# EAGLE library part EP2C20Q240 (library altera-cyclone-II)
EP2C20Q240 Auto generated by make-symbol-device-package-bsdl.ulp Rev. 19 Tip: Use split-device-symbol.ulp to generate a Device with multiple small symbols! Read HELP. Source: EP2C20Q240.BSD
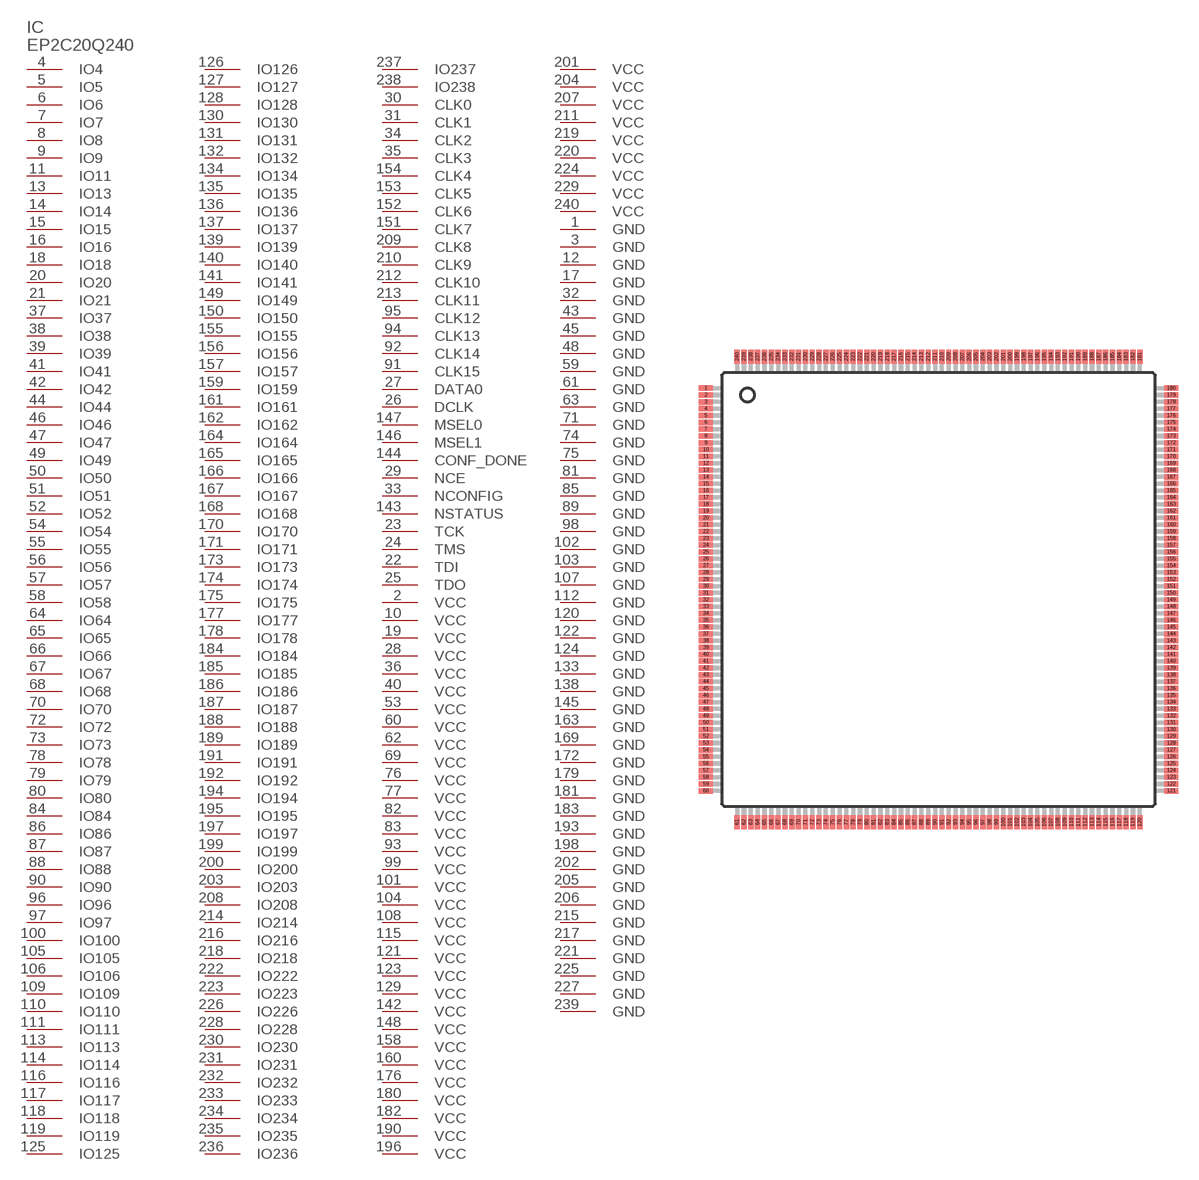
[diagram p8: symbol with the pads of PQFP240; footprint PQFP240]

Designator prefix IC

## EP2C20Q240 (MPN: EP2C20Q240C8N; OC_FARNELL: 1453472; OC_NEWARK: 51R0562)  [PQFP240]
1  GND  pwr
2  VCC  pwr
3  GND  pwr
4  IO4  out
5  IO5  out
6  IO6
7  IO7
8  IO8
9  IO9
10  VCC  pwr
11  IO11
12  GND  pwr
13  IO13
14  IO14
15  IO15
16  IO16
17  GND  pwr
18  IO18
19  VCC  pwr
20  IO20
21  IO21
22  TDI  in
23  TCK  in
24  TMS  in
25  TDO  out
26  DCLK
27  DATA0
28  VCC  pwr
29  NCE  in
30  CLK0
31  CLK1
32  GND  pwr
33  NCONFIG  in
34  CLK2
35  CLK3
36  VCC  pwr
37  IO37
38  IO38
39  IO39
40  VCC  pwr
41  IO41
42  IO42
43  GND  pwr
44  IO44
45  GND  pwr
46  IO46
47  IO47
48  GND  pwr
49  IO49
50  IO50
51  IO51
52  IO52
53  VCC  pwr
54  IO54
55  IO55
56  IO56
57  IO57
58  IO58
59  GND  pwr
60  VCC  pwr
61  GND  pwr
62  VCC  pwr
63  GND  pwr
64  IO64
65  IO65
66  IO66
67  IO67
68  IO68
69  VCC  pwr
70  IO70
71  GND  pwr
72  IO72
73  IO73
74  GND  pwr
75  GND  pwr
76  VCC  pwr
77  VCC  pwr
78  IO78
79  IO79
80  IO80
81  GND  pwr
82  VCC  pwr
83  VCC  pwr
84  IO84
85  GND  pwr
86  IO86
87  IO87
88  IO88
89  GND  pwr
90  IO90
91  CLK15
92  CLK14
93  VCC  pwr
94  CLK13
95  CLK12
96  IO96
97  IO97
98  GND  pwr
99  VCC  pwr
100  IO100
101  VCC  pwr
102  GND  pwr
103  GND  pwr
104  VCC  pwr
105  IO105
106  IO106
107  GND  pwr
108  VCC  pwr
109  IO109
110  IO110
111  IO111
112  GND  pwr
113  IO113
114  IO114
115  VCC  pwr
116  IO116
117  IO117
118  IO118
119  IO119
120  GND  pwr
121  VCC  pwr
122  GND  pwr
123  VCC  pwr
124  GND  pwr
125  IO125
126  IO126
127  IO127
128  IO128
129  VCC  pwr
130  IO130
131  IO131
132  IO132
133  GND  pwr
134  IO134
135  IO135
136  IO136
137  IO137
138  GND  pwr
139  IO139
140  IO140
141  IO141
142  VCC  pwr
143  NSTATUS  in
144  CONF_DONE  in
145  GND  pwr
146  MSEL1  in
147  MSEL0  in
148  VCC  pwr
149  IO149
150  IO150
151  CLK7
152  CLK6
153  CLK5
154  CLK4
155  IO155
156  IO156
157  IO157
158  VCC  pwr
159  IO159
160  VCC  pwr
161  IO161
162  IO162
163  GND  pwr
164  IO164
165  IO165
166  IO166
167  IO167
168  IO168
169  GND  pwr
170  IO170
171  IO171
172  GND  pwr
173  IO173
174  IO174
175  IO175
176  VCC  pwr
177  IO177
178  IO178
179  GND  pwr
180  VCC  pwr
181  GND  pwr
182  VCC  pwr
183  GND  pwr
184  IO184
185  IO185
186  IO186
187  IO187
188  IO188
189  IO189
190  VCC  pwr
191  IO191
192  IO192
193  GND  pwr
194  IO194
195  IO195
196  VCC  pwr
197  IO197
198  GND  pwr
199  IO199
200  IO200
201  VCC  pwr
202  GND  pwr
203  IO203
204  VCC  pwr
205  GND  pwr
206  GND  pwr
207  VCC  pwr
208  IO208
209  CLK8
210  CLK9
211  VCC  pwr
212  CLK10
213  CLK11
214  IO214
215  GND  pwr
216  IO216
217  GND  pwr
218  IO218
219  VCC  pwr
220  VCC  pwr
221  GND  pwr
222  IO222
223  IO223
224  VCC  pwr
225  GND  pwr
226  IO226
227  GND  pwr
228  IO228
229  VCC  pwr
230  IO230
231  IO231
232  IO232
233  IO233
234  IO234
235  IO235
236  IO236
237  IO237
238  IO238
239  GND  pwr
240  VCC  pwr

## Footprint PQFP240 (pad centres in mm)
PQFP240 Auto generated by make-symbol-device-package-bsdl.ulp Rev. 18 Source: www.altera.com .. cyc2_cii51015.pdf
smd 1 x 0.4: 1 -17.05,14.75; 2 -17.05,14.25; 3 -17.05,13.75; 4 -17.05,13.25; 5 -17.05,12.75; 6 -17.05,12.25; 7 -17.05,11.75; 8 -17.05,11.25; 9 -17.05,10.75; 10 -17.05,10.25; 11 -17.05,9.75; 12 -17.05,9.25; 13 -17.05,8.75; 14 -17.05,8.25; 15 -17.05,7.75; 16 -17.05,7.25; 17 -17.05,6.75; 18 -17.05,6.25; 19 -17.05,5.75; 20 -17.05,5.25; 21 -17.05,4.75; 22 -17.05,4.25; 23 -17.05,3.75; 24 -17.05,3.25; 25 -17.05,2.75; 26 -17.05,2.25; 27 -17.05,1.75; 28 -17.05,1.25; 29 -17.05,0.75; 30 -17.05,0.25; 31 -17.05,-0.25; 32 -17.05,-0.75; 33 -17.05,-1.25; 34 -17.05,-1.75; 35 -17.05,-2.25; 36 -17.05,-2.75; 37 -17.05,-3.25; 38 -17.05,-3.75; 39 -17.05,-4.25; 40 -17.05,-4.75; 41 -17.05,-5.25; 42 -17.05,-5.75; 43 -17.05,-6.25; 44 -17.05,-6.75; 45 -17.05,-7.25; 46 -17.05,-7.75; 47 -17.05,-8.25; 48 -17.05,-8.75; 49 -17.05,-9.25; 50 -17.05,-9.75; 51 -17.05,-10.25; 52 -17.05,-10.75; 53 -17.05,-11.25; 54 -17.05,-11.75; 55 -17.05,-12.25; 56 -17.05,-12.75; 57 -17.05,-13.25; 58 -17.05,-13.75; 59 -17.05,-14.25; 60 -17.05,-14.75; 121 17.05,-14.75; 122 17.05,-14.25; 123 17.05,-13.75; 124 17.05,-13.25; 125 17.05,-12.75; 126 17.05,-12.25; 127 17.05,-11.75; 128 17.05,-11.25; 129 17.05,-10.75; 130 17.05,-10.25; 131 17.05,-9.75; 132 17.05,-9.25; 133 17.05,-8.75; 134 17.05,-8.25; 135 17.05,-7.75; 136 17.05,-7.25; 137 17.05,-6.75; 138 17.05,-6.25; 139 17.05,-5.75; 140 17.05,-5.25; 141 17.05,-4.75; 142 17.05,-4.25; 143 17.05,-3.75; 144 17.05,-3.25; 145 17.05,-2.75; 146 17.05,-2.25; 147 17.05,-1.75; 148 17.05,-1.25; 149 17.05,-0.75; 150 17.05,-0.25; 151 17.05,0.25; 152 17.05,0.75; 153 17.05,1.25; 154 17.05,1.75; 155 17.05,2.25; 156 17.05,2.75; 157 17.05,3.25; 158 17.05,3.75; 159 17.05,4.25; 160 17.05,4.75; 161 17.05,5.25; 162 17.05,5.75; 163 17.05,6.25; 164 17.05,6.75; 165 17.05,7.25; 166 17.05,7.75; 167 17.05,8.25; 168 17.05,8.75; 169 17.05,9.25; 170 17.05,9.75; 171 17.05,10.25; 172 17.05,10.75; 173 17.05,11.25; 174 17.05,11.75; 175 17.05,12.25; 176 17.05,12.75; 177 17.05,13.25; 178 17.05,13.75; 179 17.05,14.25; 180 17.05,14.75
smd 0.4 x 1: 61 -14.75,-17.05; 62 -14.25,-17.05; 63 -13.75,-17.05; 64 -13.25,-17.05; 65 -12.75,-17.05; 66 -12.25,-17.05; 67 -11.75,-17.05; 68 -11.25,-17.05; 69 -10.75,-17.05; 70 -10.25,-17.05; 71 -9.75,-17.05; 72 -9.25,-17.05; 73 -8.75,-17.05; 74 -8.25,-17.05; 75 -7.75,-17.05; 76 -7.25,-17.05; 77 -6.75,-17.05; 78 -6.25,-17.05; 79 -5.75,-17.05; 80 -5.25,-17.05; 81 -4.75,-17.05; 82 -4.25,-17.05; 83 -3.75,-17.05; 84 -3.25,-17.05; 85 -2.75,-17.05; 86 -2.25,-17.05; 87 -1.75,-17.05; 88 -1.25,-17.05; 89 -0.75,-17.05; 90 -0.25,-17.05; 91 0.25,-17.05; 92 0.75,-17.05; 93 1.25,-17.05; 94 1.75,-17.05; 95 2.25,-17.05; 96 2.75,-17.05; 97 3.25,-17.05; 98 3.75,-17.05; 99 4.25,-17.05; 100 4.75,-17.05; 101 5.25,-17.05; 102 5.75,-17.05; 103 6.25,-17.05; 104 6.75,-17.05; 105 7.25,-17.05; 106 7.75,-17.05; 107 8.25,-17.05; 108 8.75,-17.05; 109 9.25,-17.05; 110 9.75,-17.05; 111 10.25,-17.05; 112 10.75,-17.05; 113 11.25,-17.05; 114 11.75,-17.05; 115 12.25,-17.05; 116 12.75,-17.05; 117 13.25,-17.05; 118 13.75,-17.05; 119 14.25,-17.05; 120 14.75,-17.05; 181 14.75,17.05; 182 14.25,17.05; 183 13.75,17.05; 184 13.25,17.05; 185 12.75,17.05; 186 12.25,17.05; 187 11.75,17.05; 188 11.25,17.05; 189 10.75,17.05; 190 10.25,17.05; 191 9.75,17.05; 192 9.25,17.05; 193 8.75,17.05; 194 8.25,17.05; 195 7.75,17.05; 196 7.25,17.05; 197 6.75,17.05; 198 6.25,17.05; 199 5.75,17.05; 200 5.25,17.05; 201 4.75,17.05; 202 4.25,17.05; 203 3.75,17.05; 204 3.25,17.05; 205 2.75,17.05; 206 2.25,17.05; 207 1.75,17.05; 208 1.25,17.05; 209 0.75,17.05; 210 0.25,17.05; 211 -0.25,17.05; 212 -0.75,17.05; 213 -1.25,17.05; 214 -1.75,17.05; 215 -2.25,17.05; 216 -2.75,17.05; 217 -3.25,17.05; 218 -3.75,17.05; 219 -4.25,17.05; 220 -4.75,17.05; 221 -5.25,17.05; 222 -5.75,17.05; 223 -6.25,17.05; 224 -6.75,17.05; 225 -7.25,17.05; 226 -7.75,17.05; 227 -8.25,17.05; 228 -8.75,17.05; 229 -9.25,17.05; 230 -9.75,17.05; 231 -10.25,17.05; 232 -10.75,17.05; 233 -11.25,17.05; 234 -11.75,17.05; 235 -12.25,17.05; 236 -12.75,17.05; 237 -13.25,17.05; 238 -13.75,17.05; 239 -14.25,17.05; 240 -14.75,17.05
